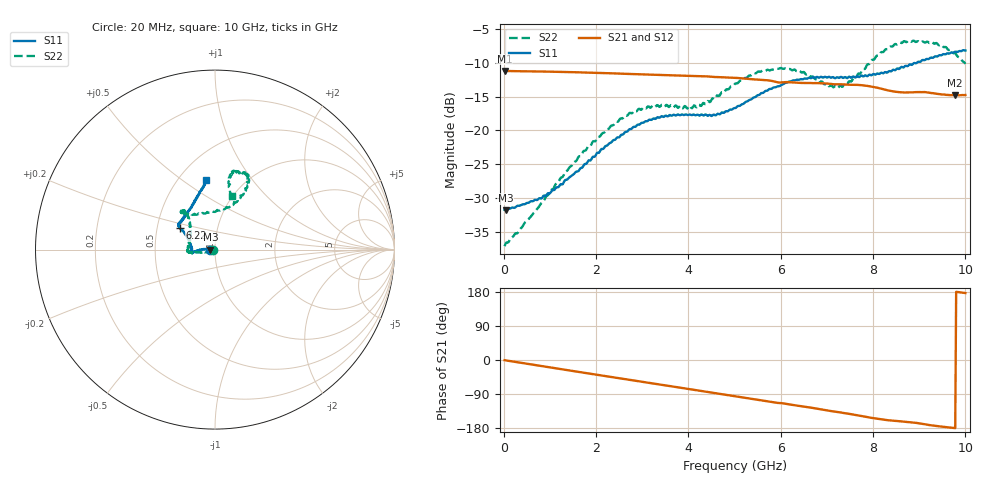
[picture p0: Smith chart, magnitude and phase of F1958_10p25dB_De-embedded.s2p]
! Integrated Device Technology
! Corporate Headquarters
! 6024 Silver Creek Valley Road
! San Jose, CA 95138  USA
! Phone:  1-408-284-8200
! Toll Free:  1-800-223-1366
! Webpage:  http://www.idt.com/
! Timing and RF Division
! 515 Groton Road, Suite 102
! Westford, MA 01886-6024
! Device:  F1958
! Description: 7-bit 0.25 dB Digital Step Attenuator
! Frequency:  0.001 -  6.000 GHz
! Package:  4x4 mm Thin QFN Plastic Package: 24 pin
! Ports:  2 RF, 12 DC
!  Pin  1  = D0
!  Pin  2  = VDD
!  Pin  3  = VMODE
!  Pin  4  = GND
!  Pin  5  = RF1  =  Port 1
!  Pin  6  = GND
!  Pin  7  = GND
!  Pin  8  = GND
!  Pin  9  = GND
!  Pin 10  = GND
!  Pin 11  = GND
!  Pin 12  = GND
!  Pin 13  = GND
!  Pin 14  = RF2  =  Port 2
!  Pin 15  = GND
!  Pin 16  = LE
!  Pin 17  = CLK
!  Pin 18  = DATA
!  Pin 19  = D6
!  Pin 20  = D5
!  Pin 21  = D4
!  Pin 22  = D3
!  Pin 23  = D2
!  Pin 24  = D1
! State:  41
! Atten State:  10.25 dB
! Voltage:  +3.30 Volts
! Current:  0.258 mA
! Data:  The device was measured on a F1958 evaluation board which has
!  individual transmission lines to the RF pins.  Data was collected
!  using a calibrated network analyzer.  The evaluation board was
!  de-embedded using Automatic Fixture Removal (AFR).
!  The reference plane is the edge of the package pin.
! Misc:
!  Action Tracker AT0419
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# GHz S dB R 50
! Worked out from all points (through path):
!   500 points, 20 MHz to 10 GHz, reference 50 ohm
!   highest |S21| = -11.20 dB at 20 MHz (marker M1); lowest = -14.8 dB at 9.78 GHz (marker M2)
!   group delay of S21, straight-line fit = 51.7 ps
!   lowest |S11| = -31.8 dB at 40 MHz (marker M3), VSWR 1.05, Z = 47.5 - j0.0681 ohm
!   |S11| at or under -10 dB: start of sweep to 8.948 GHz
!   |S22| runs from -37.1 to -6.7 dB; largest |S21 - S12| = 0.00079
!   S11 on the Smith chart (normalised r, x): 20 MHz: 0.95, -0.00; 6.22 GHz: 0.66, +0.17; 10 GHz: 0.68, +0.62
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0.02  -31.76 -178.3  -11.20 -0.5  -11.20 -0.5  -37.14 -173.0
0.04  -31.81 -178.4  -11.20 -0.9  -11.20 -0.9  -36.77 -170.0
0.8  -30.07 175.6  -11.29 -15.6  -11.29 -15.6  -30.91 -159.2
1.7  -25.52 177.3  -11.43 -32.8  -11.42 -32.8  -23.44 -167.2
2.6  -20.50 -177.2  -11.62 -49.9  -11.61 -49.9  -18.03 -173.4
2.92  -19.15 -174.4  -11.69 -56.0  -11.68 -56.1  -16.83 -174.1
3.36  -18.11 -171.9  -11.81 -64.3  -11.81 -64.4  -16.45 -176.1
4.22  -17.75 -175.6  -11.98 -80.5  -11.99 -80.6  -16.20 156.7
4.56  -17.67 177.6  -12.10 -87.0  -12.11 -87.0  -15.40 143.9
5.02  -16.69 163.8  -12.23 -95.8  -12.24 -95.8  -13.05 131.2
5.56  -14.60 152.6  -12.51 -106.0  -12.52 -106.0  -11.33 128.4
6.22  -12.76 148.4  -12.89 -117.8  -12.90 -117.8  -10.99 132.4
6.68  -12.19 145.7  -13.00 -126.2  -13.02 -126.1  -12.02 126.7
7.08  -12.19 142.1  -13.11 -134.6  -13.13 -134.5  -13.33 108.9
7.32  -12.11 139.9  -13.19 -139.0  -13.20 -138.8  -13.53 92.5
7.58  -12.03 135.7  -13.26 -143.9  -13.26 -143.9  -12.21 75.0
7.9  -11.85 127.9  -13.44 -151.2  -13.44 -151.2  -10.19 66.0
8.34  -11.25 118.5  -14.11 -159.2  -14.11 -159.2  -7.86 62.9
8.74  -10.51 111.2  -14.40 -163.3  -14.41 -163.2  -6.88 66.5
9.24  -9.27 102.4  -14.46 -172.1  -14.46 -172.1  -7.03 75.4
9.78  -8.35 98.0  -14.82 -179.8  -14.85 -179.8  -8.60 77.4
10  -8.18 97.4  -14.76 176.7  -14.80 176.8  -10.15 72.5
